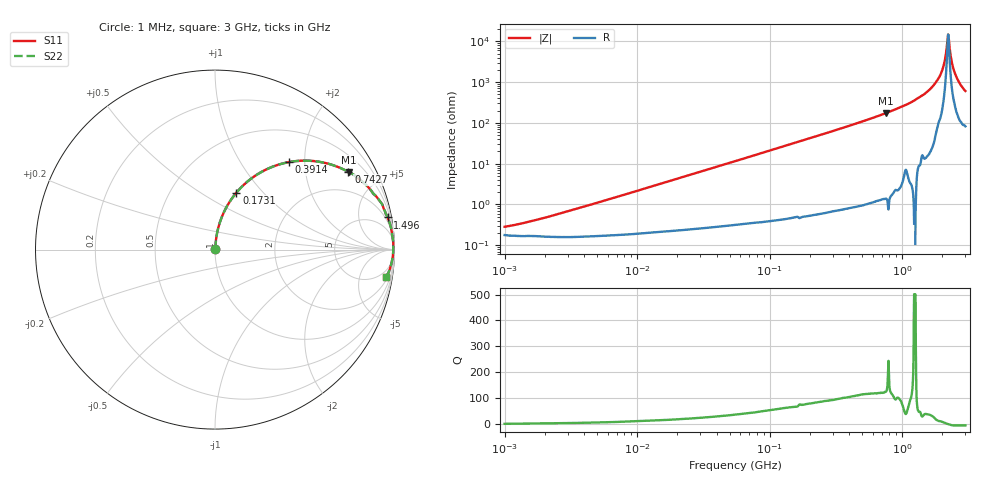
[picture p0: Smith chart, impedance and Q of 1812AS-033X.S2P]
!s-Parameter Generated by FASTRON Sdn. Bhd.
!FASTRON P/N : 1812AS-033X
!Keysight Technologies,E4991B,MY54100416,A.01.15
!Date created: Fri Oct 13 14:01:32 2023
!Version  : Rev00 Fri Oct 13 14:01:32 2023
!Data & Calibration Information:
!Freq	S11	S21	S12	S22
!PortZ  Port1:50+j0  Port2:50+j0
!When reading, reference impedance value at option line is always used.
! Remarks : This data is being provided solely for informational purposes.
# Hz S dB R 50
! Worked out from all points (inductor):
!   1601 points, 1 MHz to 3 GHz, reference 50 ohm
!   read as one part in series: L = 35.1 nH near 2.194 MHz
!   highest Q = 125 at 750.1 MHz (marker M1), where L = 36.7 nH
!   self-resonance near 2.222 GHz
!   S11 on the Smith chart (normalised r, x): 1 MHz: 1.00, +0.00; 173.1 MHz: 1.01, +0.72; 391.4 MHz: 1.02, +1.67; 742.7 MHz: 1.03, +3.42; 1.496 GHz: 1, +11; 3 GHz: 3, -12
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1000000  -50.93 51.2  -0.02 -0.1  -0.02 -0.1  -50.93 51.2
3804036  -41.43 78.5  -0.01 -0.5  -0.01 -0.5  -41.43 78.5
1.447069e7  -30.20 84.3  -0.02 -1.8  -0.02 -1.8  -30.20 84.3
5.477226e7  -18.86 81.9  -0.08 -6.5  -0.08 -6.5  -18.86 81.9
1.731398e8  -9.39 69.4  -0.57 -19.8  -0.57 -19.8  -9.39 69.4
2.083556e8  -7.99 65.8  -0.80 -23.5  -0.80 -23.5  -7.99 65.8
3.91407e8  -3.90 49.8  -2.34 -39.6  -2.34 -39.6  -3.90 49.8
7.42674e8  -1.31 30.2  -5.96 -59.3  -5.96 -59.3  -1.31 30.2
7.50144e8  -1.28 29.9  -6.04 -59.6  -6.04 -59.6  -1.28 29.9
7.925923e8  -1.12 28.2  -6.50 -61.5  -6.50 -61.5  -1.12 28.2
1.142072e9  -0.46 17.9  -10.26 -71.5  -10.26 -71.5  -0.46 17.9
1.496395e9  -0.19 10.6  -14.74 -78.0  -14.74 -78.0  -0.19 10.6
1.721456e9  -0.10 6.8  -18.48 -81.1  -18.48 -81.1  -0.10 6.8
1.931433e9  -0.07 3.9  -23.31 -81.1  -23.31 -81.1  -0.07 3.9
2.040726e9  -0.06 2.4  -27.47 -80.1  -27.47 -80.1  -0.06 2.4
2.167021e9  -0.06 0.7  -36.80 -63.6  -36.80 -63.6  -0.06 0.7
2.221924e9  -0.06 0.0  -43.46 -7.1  -43.46 -7.1  -0.06 0.0
2.278218e9  -0.06 -0.7  -37.46 57.6  -37.46 57.6  -0.06 -0.7
2.39512e9  -0.08 -2.1  -28.48 75.8  -28.48 75.8  -0.08 -2.1
2.51802e9  -0.10 -3.6  -23.97 77.6  -23.97 77.6  -0.10 -3.6
2.741597e9  -0.17 -6.3  -19.16 76.6  -19.16 76.6  -0.17 -6.3
3e9  -0.30 -9.0  -15.99 73.2  -15.99 73.2  -0.30 -9.0
